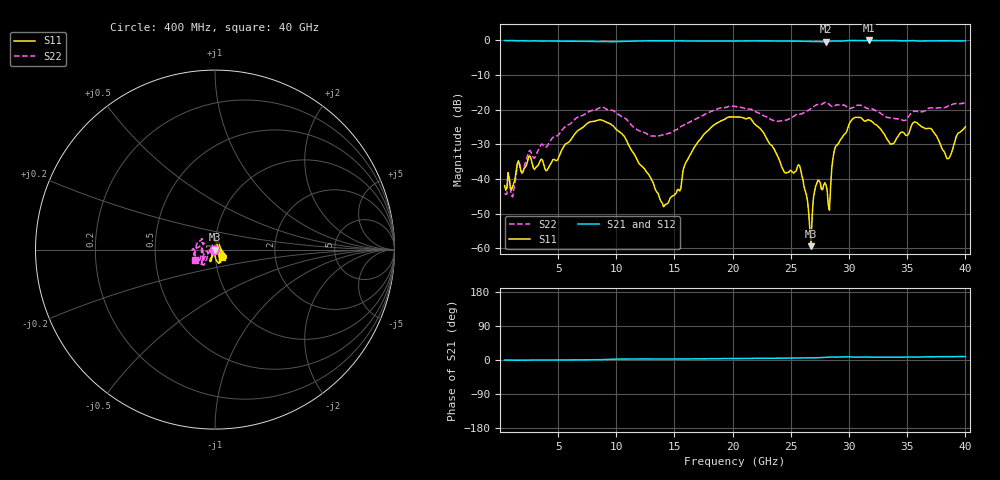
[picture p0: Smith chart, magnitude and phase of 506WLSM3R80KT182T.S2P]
!  American Technical Ceramics  Date:  8/31/2012
!  One Norden Lane
!  Huntington Station,  NY.  11746-2102
!  Tel:  (631) 622-4700  Fax:  (631) 622-4748
!  Part Number  506WLSM3R80KT182T
!  Description:  Ultra-Broadband Inductor
!  Application:  Ultra-broadband DC block decoupling, bias tee
# GHZ S DB R 50
! Freq  |S11|  S11 Ph  |S21|  S21 Ph  |S12|  S12 Ph  |S22|  S22 Ph
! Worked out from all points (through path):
!   401 points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, 400 MHz to 40 GHz, reference 50 ohm
!   highest |S21| = 0.00 dB at 31.68 GHz (marker M1); lowest = -0.4 dB at 28.02 GHz (marker M2)
!   lowest |S11| = -59.4 dB at 26.73 GHz (marker M3), VSWR 1.00, Z = 49.9 + j0.0194 ohm
!   |S11| at or under -10 dB: start of sweep to end of sweep
!   |S22| runs from -45.2 to -17.8 dB; largest |S21 - S12| = 0.005
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0.4  -41.93 -176.8  -0.04 -0.3  -0.05 -0.3  -44.12 -159.5
2.479  -33.52 149.5  -0.17 -0.3  -0.18 -0.3  -32.04 175.0
4.063  -37.43 -178.4  -0.16 -0.1  -0.16 -0.0  -30.47 -163.3
7.033  -25.34 -110.3  -0.25 0.5  -0.24 0.6  -21.74 -128.9
10.399  -26.69 -114.4  -0.29 2.5  -0.27 2.6  -21.85 -138.9
13.666  -45.03 -88.4  -0.10 2.5  -0.09 2.5  -27.50 -165.2
14.26  -47.32 -98.3  -0.11 2.6  -0.10 2.6  -27.16 -168.6
17.329  -28.02 -87.7  -0.18 3.2  -0.17 3.1  -21.82 -146.8
20.2  -22.08 -73.2  -0.17 4.2  -0.16 4.2  -19.05 -133.1
25.744  -36.15 58.9  -0.21 5.0  -0.20 4.9  -21.26 167.2
26.734  -59.41 169.5  -0.28 5.3  -0.27 5.2  -19.66 176.1
26.833  -50.52 -147.1  -0.30 5.4  -0.28 5.2  -19.42 176.9
27.229  -41.22 -158.6  -0.36 5.8  -0.35 5.6  -18.57 177.6
28.021  -41.78 -152.5  -0.38 7.3  -0.38 7.1  -17.87 -179.9
28.318  -49.02 67.4  -0.28 8.0  -0.27 8.0  -18.49 179.1
28.912  -30.33 -34.9  -0.18 7.6  -0.18 7.5  -18.57 -167.6
30.199  -23.11 -30.0  -0.01 8.0  -0.01 7.8  -19.56 -151.0
31.684  -22.94 -31.5  -0.00 7.7  -0.01 7.6  -19.75 -145.2
33.466  -29.56 6.6  -0.05 7.6  -0.06 7.4  -22.36 -171.5
35.743  -23.62 87.2  -0.13 7.5  -0.13 7.2  -20.47 140.8
38.515  -34.14 24.5  -0.10 8.6  -0.11 8.5  -18.90 -174.6
40  -24.93 -50.1  -0.13 9.0  -0.14 8.8  -17.82 -152.1
